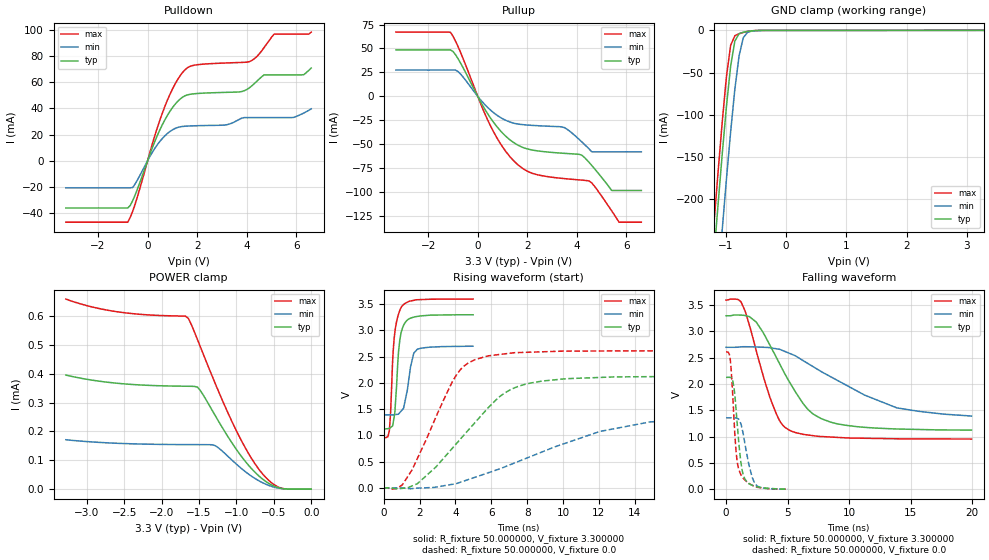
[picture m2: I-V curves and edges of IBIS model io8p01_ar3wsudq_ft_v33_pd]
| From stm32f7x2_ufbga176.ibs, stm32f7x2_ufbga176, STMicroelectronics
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|   Model io8p01_ar3wsudq_ft_v33_pd
[Model]  io8p01_ar3wsudq_ft_v33_pd
Model_type I/O
Polarity   Non-Inverting
Enable   Active-Low
Vinl =   0.990000V
Vinh =   2.310000V
Vmeas =  1.650000V
Cref =   50.000000pF
Rref =   100.000000M
Vref =   0.0V
C_comp   3.857500pF   3.760500pF   3.941700pF
[Temperature Range]   25.000000   0.125000k   -40.000000
[Pullup Reference]   3.300000V   2.700000V   3.600000V
[Pulldown Reference]   0.0V   0.0V   0.0V
[POWER Clamp Reference]   3.300000V   2.700000V   3.600000V
[GND Clamp Reference]   0.0V   0.0V   0.0V
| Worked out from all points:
|   slope of the pulldown table from 0 to 0.495 V, typ, clamps not added: 20.9 ohm
|   slope of the pullup table from 0 to 0.495 V, typ, clamps not added: 22.6 ohm
|   GND clamp passes 1 mA (typ) near -0.62 V on its own axis
|   rising waveform, R_fixture 50.000000, V_fixture 3.300000: 20-80 % time 277ps typ, 398ps min, 275ps max; typ from 1.12 V to 3.3 V
|   rising waveform, R_fixture 50.000000, V_fixture 0.0: 20-80 % time 3.36ns typ, 6.53ns min, 2.12ns max; typ from 0 V to 2.13 V
|   falling waveform, R_fixture 50.000000, V_fixture 3.300000: 20-80 % time 3.22ns typ, 6.41ns min, 2.04ns max; typ from 3.3 V to 1.12 V
|   falling waveform, R_fixture 50.000000, V_fixture 0.0: 20-80 % time 515ps typ, 709ps min, 442ps max; typ from 2.13 V to 0 V
[Pulldown]
|Voltage   I(typ)   I(min)   I(max)
-3.3V     -36.18mA   -20.77mA   -47.07mA
-800mV    -36.18mA   -20.77mA   -47.07mA
-600mV    -30.5mA    -20.52mA   -38.69mA
700mV     31.4mA     19.11mA    41.71mA
1.2V      45.15mA    25.37mA    61.75mA
1.6V      50.35mA    26.5mA     71.06mA
3.1V      52.27mA    27.26mA    74.75mA
4.1V      55.7mA     32.99mA    75.8mA
4.7V      65.71mA    32.99mA    86.63mA
5.1V      65.71mA    32.99mA    96.88mA
6.3V      65.85mA    36.49mA    96.88mA
6.6V      70.9mA     39.7mA     98.44mA
[Pullup]
|Voltage   I(typ)   I(min)   I(max)
-3.3V     48.5mA     27.43mA    67.09mA
-1.1V     48.5mA     27.43mA    66.83mA
-700mV    35.12mA    23.48mA    46.33mA
500mV     -22.07mA   -14mA      -30.03mA
1.5V      -49.1mA    -28.3mA    -68.56mA
2.2V      -56.04mA   -30.32mA   -80.35mA
3.5V      -59.53mA   -32.72mA   -85.92mA
4.2V      -61.52mA   -47.6mA    -87.46mA
4.5V      -69.21mA   -55.15mA   -88.44mA
5.4V      -98.3mA    -57.9mA    -119.4mA
5.7V      -98.3mA    -57.9mA    -131.4mA
6.6V      -98.3mA    -57.9mA    -131.4mA
[GND_clamp]
|Voltage   I(typ)   I(min)   I(max)
-3.3V     -2.332A    -2.407A    -2.312A
-1.2V     -270.2mA   -361.4mA   -232.1mA
-1.13V    -207.3mA   -298.1mA   -169mA
-1.06V    -146.7mA   -236.2mA   -108.8mA
-990mV    -90.18mA   -176.4mA   -54.97mA
-920mV    -42.21mA   -120mA     -17.69mA
-850mV    -12.58mA   -69.47mA   -6.279mA
-780mV    -3.983mA   -30.01mA   -3.9mA
-710mV    -2.112mA   -8.623mA   -2.396mA
-640mV    -1.159mA   -2.292mA   -1.234mA
-570mV    -535.1uA   -830.5uA   -490.2uA
3.28V     81.28uA    57.87uA    93.98uA
[POWER_clamp]
|Voltage   I(typ)   I(min)   I(max)
-3.28V    395.3uA    171.3uA    658.7uA
-2.6V     367.1uA    159uA      614.9uA
-1.68V    356.7uA    154.4uA    599.4uA
-1.64V    356.5uA    154.4uA    590.8uA
-1.52V    353.6uA    154.3uA    518.3uA
-1.48V    341.1uA    154.2uA    492.3uA
-1.28V    253.6uA    150.4uA    364.2uA
-960mV    123.1uA    77.55uA    181.6uA
-720mV    50.52uA    32.03uA    76.18uA
-560mV    18.94uA    12.27uA    28.65uA
-440mV    5.104uA    3.69uA     7.327uA
0V        0A         0A         0A
[Ramp]
| variable   typ   min   max
dV/dt_r  1.27692/3.35591n   0.80010/6.63201n   1.56630/2.11388n
dV/dt_f  1.30254/3.22804n   0.74298/6.40329n   1.58743/2.03762n
R_load = 50.000000
[Rising Waveform]
R_fixture= 50.000000
V_fixture= 3.300000
V_fixture_min= 2.700000
V_fixture_max= 3.600000
|time   V(typ)   V(min)   V(max)
0s        1.123V     1.391V     953.8mV
320.3ps   1.131V     1.39V      1.099V
390.4ps   1.15V      1.39V      1.455V
510.5ps   1.199V     1.391V     2.476V
650.7ps   1.577V     1.396V     3.034V
830.8ps   2.593V     1.408V     3.313V
991ps     2.978V     1.469V     3.446V
1.682ns   3.253V     2.569V     3.574V
1.882ns   3.267V     2.642V     3.585V
4.985ns   3.299V     2.699V     3.598V
[Rising Waveform]
R_fixture= 50.000000
V_fixture= 0.0
V_fixture_min= 0.0
V_fixture_max= 0.0
|time   V(typ)   V(min)   V(max)
0s        196.8uV    83.41uV    722.1uV
1.041ns   -10.13mV   -4.317mV   56.19mV
1.882ns   78.87mV    -5.01mV    561mV
3.844ns   759.4mV    67.51mV    2.03V
5.085ns   1.24V      200.2mV    2.442V
6.607ns   1.774V     378.9mV    2.548V
8.208ns   1.998V     598.2mV    2.586V
12.05ns   2.104V     1.074V     2.608V
14.77ns   2.119V     1.251V     2.611V
19.94ns   2.127V     1.358V     2.611V
[Falling Waveform]
R_fixture= 50.000000
V_fixture= 3.300000
V_fixture_min= 2.700000
V_fixture_max= 3.600000
|time   V(typ)   V(min)   V(max)
0s        3.299V     2.699V     3.598V
1.201ns   3.311V     2.707V     3.568V
2.442ns   3.181V     2.705V     2.643V
3.604ns   2.721V     2.688V     1.721V
4.324ns   2.398V     2.662V     1.313V
5.085ns   2.064V     2.59V      1.129V
6.647ns   1.518V     2.391V     1.031V
8.488ns   1.275V     2.14V      992.2mV
13.89ns   1.144V     1.545V     958.2mV
19.94ns   1.123V     1.391V     953.8mV
[Falling Waveform]
R_fixture= 50.000000
V_fixture= 0.0
V_fixture_min= 0.0
V_fixture_max= 0.0
|time   V(typ)   V(min)   V(max)
0s        2.127V     1.358V     2.611V
340.3ps   2.124V     1.357V     2.473V
500.5ps   2.081V     1.357V     1.968V
640.6ps   1.939V     1.357V     1.359V
880.9ps   1.32V      1.347V     569.5mV
1.181ns   553.9mV    1.256V     287.8mV
1.512ns   203.8mV    892.7mV    179.5mV
1.842ns   108.4mV    481.6mV    110mV
2.312ns   58.39mV    120.4mV    51.8mV
4.985ns   196.8uV    83.41uV    722.1uV
